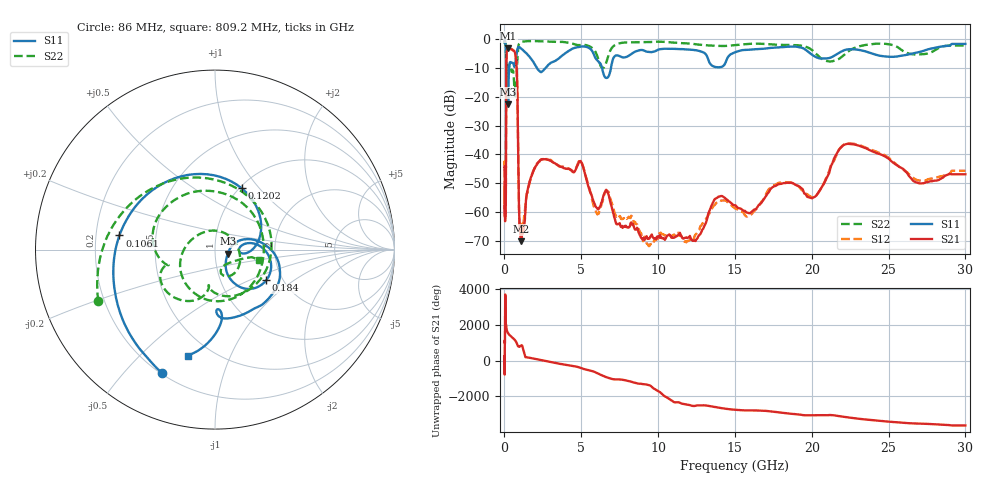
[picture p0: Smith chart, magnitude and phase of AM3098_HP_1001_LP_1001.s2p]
! Date/Time: Thu, Feb 28, 2019 8:41 AM
! Network Analyzer: Agilent Technologies E8364B Rev: A.07.50.67
! Sweep from 0.010 to 30.000 GHz, 1601 Points, Sweep Type: LOG
! Power Supply: 5.022 V, 0.002 A
# Hz S DB R 50
!freq MagS11 AngS11 MagS21 AngS21 MagS12 AngS12 MagS22 AngS22
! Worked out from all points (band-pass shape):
!   1601 points, 10 MHz to 30 GHz, reference 50 ohm
!   highest |S21| = -3.05 dB at 258.6 MHz (marker M1); lowest = -70.2 dB at 1.06 GHz (marker M2)
!   |S21| within 3 dB of the highest: 130.2 MHz to 735.5 MHz (605.3 MHz wide, 140 % of centre)
!   lowest |S11| = -22.5 dB at 239.9 MHz (marker M3), VSWR 1.16, Z = 57.6 - j2.57 ohm
!   |S11| at or under -10 dB: 191.3 MHz to 302.9 MHz (111.6 MHz wide, 45.2 % of centre); 2.12 GHz to 2.665 GHz (545.7 MHz wide, 22.8 % of centre); 6.358 GHz to 6.929 GHz (571.6 MHz wide, 8.6 % of centre)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
!   |S22| runs from -19.8 to -0.5 dB; largest |S21 - S12| = 0.011
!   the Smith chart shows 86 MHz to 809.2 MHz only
!   S11 on the Smith chart (normalised r, x): 86 MHz: 0.20, -0.64; 106.1 MHz: 0.30, +0.07; 120.2 MHz: 1.03, +0.81; 184 MHz: 1.65, -0.63; 809.2 MHz: 0.38, -0.70
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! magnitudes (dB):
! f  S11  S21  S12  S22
! 10 MHz  -0.3  -44.2  -44.2  -0.6
! 38.04 MHz  -0.5  -60.2  -59.7  -0.9
! 51.36 MHz  -0.8  -48.2  -48.8  -1.3
! 86 MHz  -2.5  -55.4  -55.8  -3.0
! 106.1 MHz  -5.4  -28.6  -28.5  -6.9
! 120.2 MHz  -8.6  -10.9  -10.8  -10.3
! 144.7 MHz  -17.2  -4.3  -4.3  -13.4
! 184 MHz  -9.6  -3.6  -3.6  -8.9
! 239.9 MHz  -22.5  -3.1  -3.0  -11.3
! 258.6 MHz  -17.2  -3.0  -3.0  -10.8
! 550.5 MHz  -8.2  -3.8  -3.7  -10.8
! 809.2 MHz  -4.3  -11.8  -11.8  -11.9
! 954.5 MHz  -2.6  -60.0  -60.1  -1.5
! 1.06 GHz  -3.0  -70.2  -65.6  -0.9
! 2.084 GHz  -9.6  -43.7  -43.4  -0.6
! 4.952 GHz  -2.5  -42.3  -42.2  -1.9
! 7.926 GHz  -6.1  -65.3  -62.1  -1.0
! 12.07 GHz  -3.5  -68.3  -69.8  -1.4
! 13.95 GHz  -9.7  -54.6  -56.3  -2.2
! 20.1 GHz  -5.6  -55.0  -54.9  -4.0
! 22.67 GHz  -3.4  -36.5  -36.3  -3.2
! 30 GHz  -1.5  -46.9  -45.7  -2.1
